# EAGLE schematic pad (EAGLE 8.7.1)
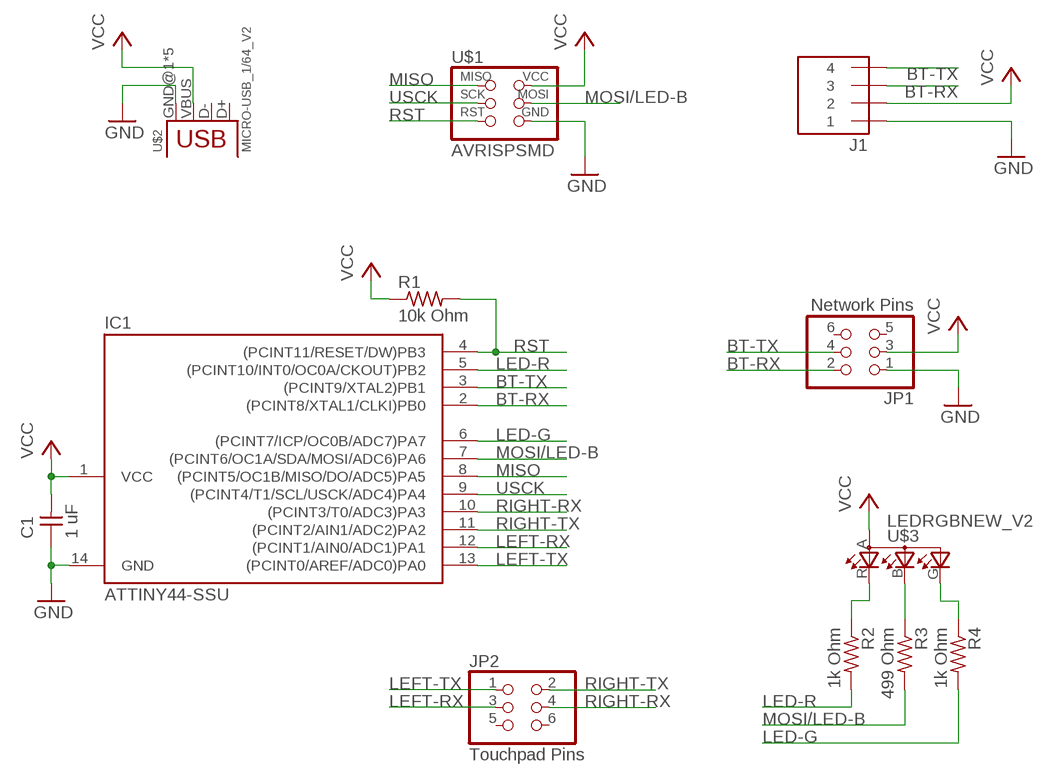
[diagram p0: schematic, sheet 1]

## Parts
C1  1 uF  CAP-UNPOLARIZEDFAB  [C1206FAB]
IC1  ATTINY44-SSU  [SOIC14]
J1  PIN_HEADER_SMD_1X4  [1X04SMD]
JP1  Network Pins  PIN_HEADER_SMD_2X3  [2X03SMD]
JP2  Touchpad Pins  PIN_HEADER_SMD_2X3  [2X03SMD]
R1  10k Ohm  RESISTOR1206FAB  [R1206FAB]
R2  1k Ohm  RESISTOR1206FAB  [R1206FAB]
R3  499 Ohm  RESISTOR1206FAB  [R1206FAB]
R4  1k Ohm  RESISTOR1206FAB  [R1206FAB]
U$1  AVRISPSMD  [2X03SMD]
U$2  MICRO-USB_1/64_V2  [DX4R005HJ5_64_V2]
U$3  LEDRGBNEW_V2  [P-LCC-4-3_V2]

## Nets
BT-RX: IC1.2((PCINT8/XTAL1/CLKI)PB0) J1.3 JP1.2
BT-TX: IC1.3((PCINT9/XTAL2)PB1) J1.4 JP1.4
GND: C1.1 IC1.14(GND) J1.1 JP1.1 U$1.6(GND) U$2.GND@1(GND) U$2.GND@2(GND) U$2.GND@3(GND) U$2.GND@4(GND) U$2.GND@5(GND)
LED-G: IC1.6((PCINT7/ICP/OC0B/ADC7)PA7) R4.2
LED-R: IC1.5((PCINT10/INT0/OC0A/CKOUT)PB2) R2.2
LEFT-RX: IC1.12((PCINT1/AIN0/ADC1)PA1) JP2.3
LEFT-TX: IC1.13((PCINT0/AREF/ADC0)PA0) JP2.1
MISO: IC1.8((PCINT5/OC1B/MISO/DO/ADC5)PA5) U$1.1(MISO)
MOSI/LED-B: IC1.7((PCINT6/OC1A/SDA/MOSI/ADC6)PA6) R3.2 U$1.4(MOSI)
N$1: R3.1 U$3.B(CBLUE)
N$2: R2.1 U$3.R(CRED)
N$3: R4.1 U$3.G(CGREEN)
RIGHT-RX: IC1.10((PCINT3/T0/ADC3)PA3) JP2.4
RIGHT-TX: IC1.11((PCINT2/AIN1/ADC2)PA2) JP2.2
RST: IC1.4((PCINT11/RESET/DW)PB3) R1.2 U$1.5(RST)
USCK: IC1.9((PCINT4/T1/SCL/USCK/ADC4)PA4) U$1.3(SCK)
VCC: C1.2 IC1.1(VCC) J1.2 JP1.3 R1.1 U$1.2(VCC) U$2.VBUS U$3.A(A2)
Unconnected: JP1.5 JP1.6 JP2.5 JP2.6 U$2.D+ U$2.D-

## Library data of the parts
C1 = fab:CAP-UNPOLARIZED
IC1 = fab:ATTINY44
J1 = fab:PIN_HEADER_SMD_1X4
JP1 JP2 = fab:PIN_HEADER_SMD_2X3: PIN HEADER
R1-R4 = fab:RESISTOR: Resistor (US Symbol)
U$1 = fab:AVRISP
U$2 = fab:MICRO-USB: SMD micro USB connector as found in the fablab inventory. Three footprint variants included: original, as described by manufacturer's datasheet for milling with the 1/100" bit for milling with the 1/64" bit Made by Zaerc.
U$3 = fab:LEDRGBNEW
